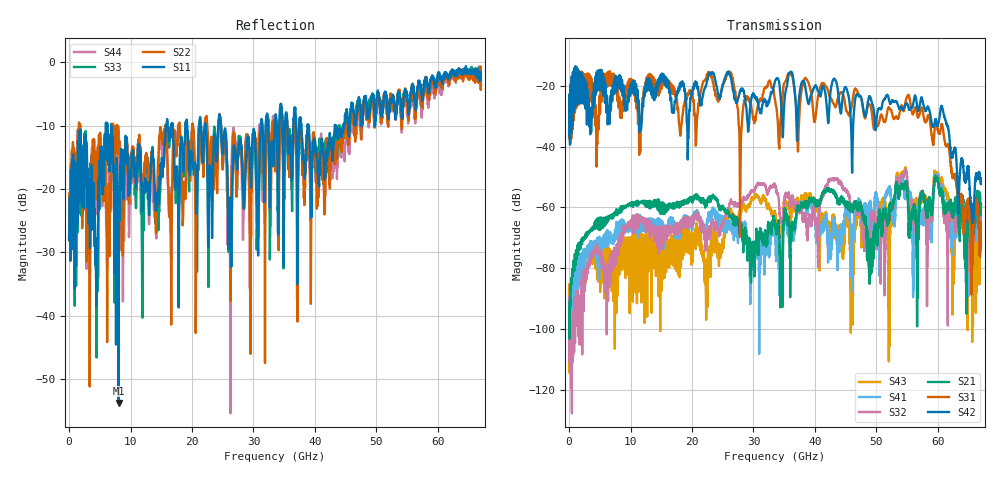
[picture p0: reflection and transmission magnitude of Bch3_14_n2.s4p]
!Agilent Technologies,N5247A,US51170199,A.09.90.13
!Agilent N5247A: A.09.90.13
!Date: Wednesday, October 17, 2018 18:08:53
!Correction: S11(Full 4 Port(1,2,3,4))
!S12(Full 4 Port(1,2,3,4))
!S13(Full 4 Port(1,2,3,4))
!S14(Full 4 Port(1,2,3,4))
!S21(Full 4 Port(1,2,3,4))
!S22(Full 4 Port(1,2,3,4))
!S23(Full 4 Port(1,2,3,4))
!S24(Full 4 Port(1,2,3,4))
!S31(Full 4 Port(1,2,3,4))
!S32(Full 4 Port(1,2,3,4))
!S33(Full 4 Port(1,2,3,4))
!S34(Full 4 Port(1,2,3,4))
!S41(Full 4 Port(1,2,3,4))
!S42(Full 4 Port(1,2,3,4))
!S43(Full 4 Port(1,2,3,4))
!S44(Full 4 Port(1,2,3,4))
!S4P File: Measurements: <S11,S12,S13,S14>,
!<S21,S22,S23,S24>,
!<S31,S32,S33,S34>,
!<S41,S42,S43,S44>:
# Hz S  dB  R 50
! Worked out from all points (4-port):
!   6701 points, 10 MHz to 67 GHz, reference 50 ohm
!   strongest paths, dB at 10 MHz, 16.76 GHz, 33.51 GHz, 50.25 GHz, 67 GHz:
!     S42: -36.5, -28.7, -18.5, -27.9, -51.8
!     S31: -37.2, -21.4, -24.5, -33.1, -71.6
!     S21: -96.9, -60.1, -65.7, -66.3, -58.7
!     S32: -94.5, -66.5, -52.9, -61.7, -68.0
!     S41: -89.5, -67.3, -69.8, -60.5, -73.3
!     S43: -85.4, -78.0, -61.8, -58.6, -67.4
!   lowest |S11| = -53.8 dB at 8.059 GHz (marker M1), VSWR 1.00, Z = 49.8 + j0.0836 ohm
!   |S11| at or under -10 dB: start of sweep to 5.98 GHz; 6.225 GHz to 15.74 GHz (9.513 GHz wide, 86.6 % of centre); 24.71 GHz to 31.16 GHz (6.449 GHz wide, 23.1 % of centre)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
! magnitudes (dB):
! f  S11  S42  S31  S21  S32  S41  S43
! 10 MHz  -28.0  -36.5  -37.2  -96.9  -94.5  -89.5  -85.4
! 8.059 GHz  -53.8  -19.3  -27.2  -61.7  -74.0  -69.2  -71.8
! 34.5 GHz  -6.7  -25.9  -28.3  -78.6  -64.6  -74.1  -67.2
! 39.13 GHz  -12.3  -24.8  -20.0  -57.9  -62.8  -58.2  -55.8
! 45.99 GHz  -6.5  -41.7  -26.4  -60.7  -59.6  -76.2  -79.8
! 55.15 GHz  -6.7  -26.6  -23.1  -59.9  -53.5  -54.9  -56.9
! 67 GHz  -2.7  -51.8  -71.6  -58.7  -68.0  -73.3  -67.4
